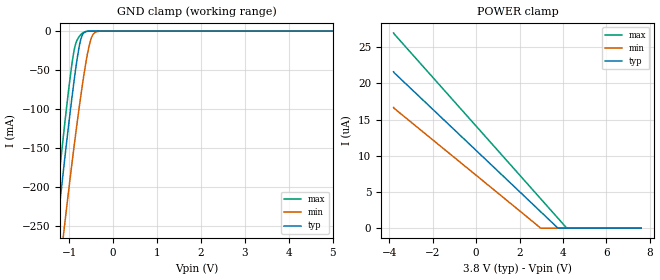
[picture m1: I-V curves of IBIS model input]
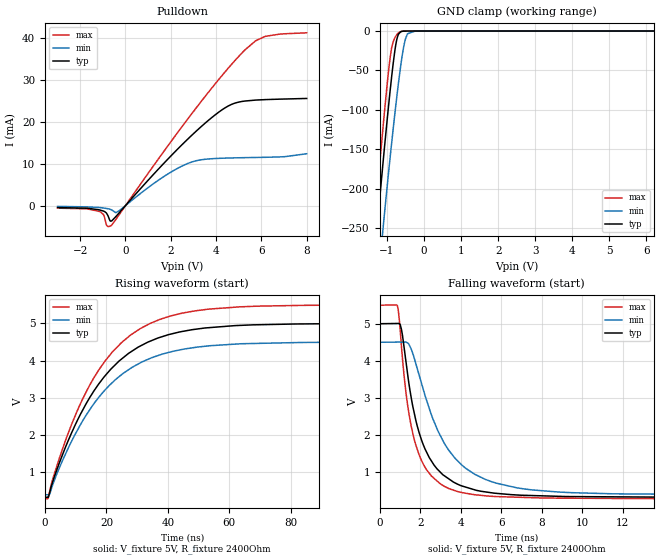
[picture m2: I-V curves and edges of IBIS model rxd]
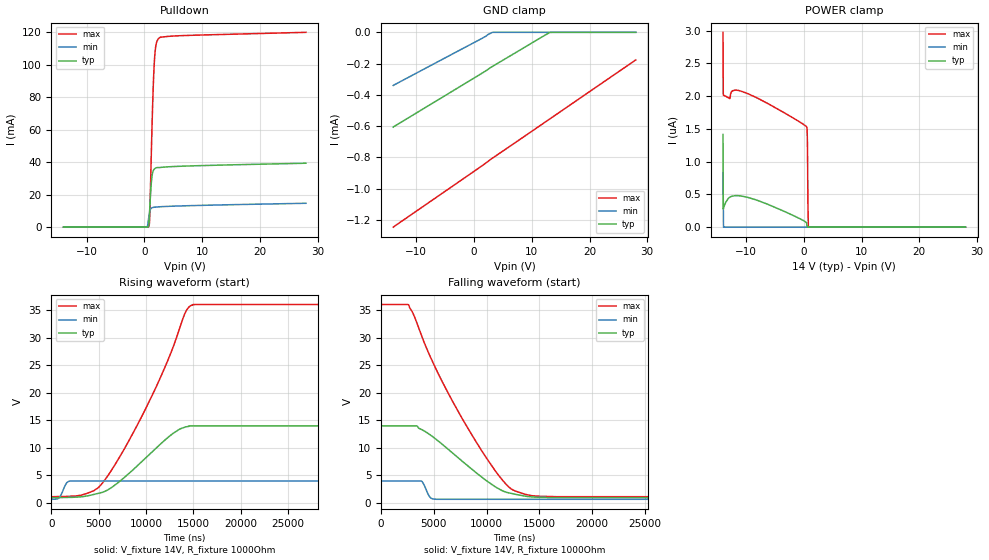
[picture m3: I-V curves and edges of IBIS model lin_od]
|Texas Instruments Incorporated
|TLIN1022-Q1 Dual Local Interconnect Network (LIN) Transceiver with Dominant
| State Timeout
[IBIS Ver]   4.1
[File name]   tlin1022-q1.ibs
[Date]   01/05/2018
[File Rev]   1.0
[Source]
| Texas Instruments Incorporated.
| Analog-eLab Design Center, HPA
| 12500 TI Blvd
| Dallas, TX -75243
[Notes]
| Rev 1.0: 01/05/2018
| - Initial version of the model
| - Model generated from simulations in SPECTRE
| - Model matched to SPICE simulation
| - C_comp although listed in numerical order of value are
|   obtained from varying PVT conditions. For PVT conditions for
|   each specific value refer the buffer description under
|   respective [Model]. IBIS model user is responsible for using
|   appropriate C_comp to simulate for Signal Integrity.
| - Warnings regarding combined Non-monotonicity of various models
|   have been reviewed and considered minor and can be ignored.
| - slow corner of lin_output model correlated for frequencies from 2KHz to 10KHz
[Disclaimer]
| This model is designed as an aid for customers of Texas Instruments.
| TI and its licensors and suppliers make no warranties, either expressed
| or implied, with respect to this  model, including the warranties of
| merchantability or fitness for a particular purpose. The model is
| provided solely on an "as is" basis. The entire risk as to its quality
| and performance is with the customer.
[Copyright]
(C) Copyright 2018 Texas Instruments Incorporated.All rights reserved.
|  Component TLIN1022DRQ1 14-pin SOIC - D package
|  Part # TLIN1022DRQ1
[Component]   TLIN1022DRQ1
[Manufacturer]  TI
[Package]   |14 SOIC - D package
|   typ   min   max
R_pkg   0.1   0.08   0.12
L_pkg   1.0nH   0.8nH   1.2nH
C_pkg   0.2pF   0.16pF   0.24pF
[Pin]  signal_name model_name   R_pin   L_pin   C_pin
1   RXD1   rxd   NA   NA   NA
2   EN1   input   NA   NA   NA
3   TXD1   input   NA   NA   NA
4   RXD2   rxd   NA   NA   NA
5   EN2   input   NA   NA   NA
6   NC   nc   NA   NA   NA
7   TXD2   input   NA   NA   NA
8   GND   gnd   NA   NA   NA
9   LIN2   lin   NA   NA   NA
10   VSUP   power   NA   NA   NA
11   NC   nc   NA   NA   NA
12   NC   nc   NA   NA   NA
13   LIN1   lin   NA   NA   NA
14   NC   nc   NA   NA   NA
|  Component TLIN1022DMTRQ1 14-pin VSON - DMT package
|  Part # TLIN1022DMTRQ1
[Component]   TLIN1022DMTRQ1
[Manufacturer]  TI
[Package]   |14 VSON - DMT package
|   typ   min   max
R_pkg   0   0   0
L_pkg   0   0   0
C_pkg   0   0   0
[Pin]  signal_name model_name   R_pin   L_pin   C_pin
1   RXD1   rxd   NA   NA   NA
2   EN1   input   NA   NA   NA
3   TXD1   input   NA   NA   NA
4   RXD2   rxd   NA   NA   NA
5   EN2   input   NA   NA   NA
6   NC   nc   NA   NA   NA
7   TXD2   input   NA   NA   NA
8   GND   gnd   NA   NA   NA
9   LIN2   lin   NA   NA   NA
10   VSUP   power   NA   NA   NA
11   NC   nc   NA   NA   NA
12   NC   nc   NA   NA   NA
13   LIN1   lin   NA   NA   NA
14   NC   nc   NA   NA   NA
|   Model Selectors
[Model Selector] lin
lin_od   14.0V   digital I/O_open_drain
lin_output   14.0V   digital Output
| Models and submodels in the file (4): input (Input), rxd (Open_sink), lin_od (I/O_open_drain), lin_output (Output)
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|   input Model
[Model]   input
Model_type   Input
Vinl = 0.8
Vinh = 2
|   typ   min   max
C_comp   3.46465E-12   3.07372E-12   4.01486E-12
| Where Nom  PVT is Nominal Process, 3.8V, 27C
|   Fast PVT is Strong Process,  4.2V, -55C
|   Slow PVT is Weak Process,   3V, 165C
[Voltage Range]   3.8   3   4.2
|Junction Temperature
[Temperature Range]   27   165   -55
[Power Clamp Reference]   3.8   3   4.2
[GND Clamp Reference]   0   0   0
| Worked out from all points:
|   GND clamp passes 1 mA (typ) near -0.63 V on its own axis
[GND Clamp]
|   Voltage   I(typ)   I(min)   I(max)
-3.8V     -1.716A    -1.741A    -1.714A
-1.417V   -329.7mA   -408.3mA   -288.7mA
-1.292V   -261.7mA   -342.8mA   -218.9mA
-1.269V   -249.6mA   -331mA     -206.5mA
-1.11V    -167.2mA   -250.8mA   -122.4mA
-904.4mV  -70.09mA   -154.5mA   -29.5mA
-847.4mV  -46.14mA   -129.4mA   -15.27mA
-767.6mV  -18.24mA   -95.69mA   -6.643mA
-665mV    -2.116mA   -55.77mA   -1.406mA
-494mV    -29.94uA   -8.423mA   -15.55uA
-300.2mV  -812.1nA   -88.71uA   -911.7nA
7.6V      0A         0A         0A
[POWER Clamp]
|   Voltage   I(typ)   I(min)   I(max)
-3.8V     21.6uA     16.67uA    26.97uA
2.96V     2.302uA    13.73nA    4.1uA
3.758V    23.08nA    0A         1.408uA
4.169V    0A         0A         15.11nA
7.6V      0A         0A         0A
|   rxd Model
[Model]   rxd
Model_type   Open_sink
Polarity   Non-Inverting
Vmeas = 2.5
Vref = 5
Cref = 2pF
Rref = 2400
|   typ   min   max
C_comp   3.72956E-12   3.27827E-12   4.2623E-12
| Where Nom  PVT is Nominal Process, 5V, 27C
|   Fast PVT is Strong Process,  5.5V, -55C
|   Slow PVT is Weak Process,   4.5V, 165C
[Voltage Range]   5   4.5   5.5
|Junction Temperature
[Temperature Range]   27   165   -55
[Pullup Reference]   5   4.5   5.5
[Pulldown Reference]   0   0   -0
[Power Clamp Reference]   5   4.5   5.5
[GND Clamp Reference]   0   0   0
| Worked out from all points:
|   slope of the pulldown table from 0 to 0.75 V, typ, clamps not added: 164 ohm
|   GND clamp passes 1 mA (typ) near -0.63 V on its own axis
|   falling waveform, V_fixture 5V, R_fixture 2400Ohm: 20-80 % time 1.33ns typ, 2.1ns min, 989ps max; typ from 5 V to 0.318 V
|   rising waveform, V_fixture 5V, R_fixture 2400Ohm: 20-80 % time 20.5ns typ, 20.7ns min, 20.1ns max; typ from 0.318 V to 5 V
[Pulldown]
|   Voltage   I(typ)   I(min)   I(max)
-3V       -478.7uA   -191.2uA   -603.9uA
-1.174V   -992.2uA   -450.9uA   -1.367mA
-965mV    -1.321mA   -581.3uA   -2.223mA
-844mV    -1.756mA   -677uA     -4.594mA
-646mV    -3.719mA   -938.5uA   -4.804mA
-426mV    -2.622mA   -1.694mA   -3.306mA
1.51V     9.031mA    6.263mA    11.55mA
2.841V    16.32mA    10.23mA    21.3mA
4.381V    23.25mA    11.31mA    31.77mA
5.283V    24.93mA    11.43mA    37.15mA
6.174V    25.26mA    11.51mA    40.34mA
8V        25.54mA    12.36mA    41.18mA
[GND Clamp]
|   Voltage   I(typ)   I(min)   I(max)
-3V       -1.245A    -1.286A    -1.23A
-1.559V   -408.7mA   -484.2mA   -369.9mA
-1.284V   -257.7mA   -339mA     -214.7mA
-1.086V   -155.7mA   -239.7mA   -110.7mA
-910mV    -72.76mA   -157.3mA   -31.65mA
-833mV    -40.68mA   -123.5mA   -13.39mA
-767mV    -18.25mA   -95.75mA   -6.8mA
-635mV    -1.061mA   -45.43mA   -766.8uA
-536mV    -90.64uA   -16.53mA   -55.21uA
-448mV    -8.124uA   -3.48mA    -2.688uA
-239mV    0A         -18.54uA   0A
8V        0A         0A         0A
[POWER Clamp]
|   Voltage   I(typ)   I(min)   I(max)
-3V       0A         0A         0A
0V        0A         0A         0A
8V        0A         0A         0A
[Ramp]
R_load = 2400
|   typ   min   max
dV/dt_r   2.80934/2.05464e-08   2.46843/2.06734e-08   3.13188/2.01086e-08
dV/dt_f   2.80935/1.32286e-09   2.46843/2.098e-09   3.13188/9.89047e-10
[Falling Waveform]
V_fixture = 5V
V_fixture_min = 4.5V
V_fixture_max = 5.5V
R_fixture = 2400Ohm
C_fixture = 0F
|   Time   V(typ)   V(min)   V(max)
0s        5V         4.5V       5.5V
877.3ps   5.007V     4.505V     5.486V
1.073ns   4.858V     4.506V     4.422V
1.389ns   3.611V     4.479V     2.779V
2.02ns    1.942V     3.48V      1.367V
2.871ns   1.064V     2.115V     740.3mV
4.079ns   620.7mV    1.177V     442.5mV
5.756ns   424.7mV    699.4mV    337.5mV
9.477ns   337.3mV    442.6mV    293.3mV
40ns      317.8mV    385.9mV    280.2mV
[Rising Waveform]
V_fixture = 5V
V_fixture_min = 4.5V
V_fixture_max = 5.5V
R_fixture = 2400Ohm
C_fixture = 0F
|   Time   V(typ)   V(min)   V(max)
0s        317.8mV    385.9mV    280.2mV
943.3ps   319.6mV    384.8mV    279.9mV
1.502ns   449.3mV    398.4mV    480.9mV
6.576ns   1.653V     1.468V     1.83V
11.47ns   2.545V     2.266V     2.829V
15.68ns   3.152V     2.812V     3.505V
21.94ns   3.811V     3.409V     4.233V
34.19ns   4.521V     4.058V     5V
53.07ns   4.885V     4.395V     5.385V
600ns     5V         4.5V       5.5V
|   lin_od Model
[Model]   lin_od
Model_type   I/O_open_drain
Polarity   Non-Inverting
Enable   Active-High
Vinl = 5.6
Vinh = 8.4
Vmeas = 7
Vref = 14
Cref = 2pF
Rref = 1000
|   typ   min   max
C_comp   3.52891E-11   3.03138E-11   3.67824E-11
[Model spec]
|subparameter
Vinl   5.6   1.6   14.4
Vinh   8.4   2.4   21.6
| Where Nom  PVT is Nominal Process, 14V, 27C
|   Fast PVT is Strong Process,  36V, -55C
|   Slow PVT is Weak Process,   4V, 165C
[Voltage Range]   14   4   36
|Junction Temperature
[Temperature Range]   27   165   -55
[Pullup Reference]   14   4   36
[Pulldown Reference]   -0   0   0
[Power Clamp Reference]   14   4   36
[GND Clamp Reference]   0   0   0
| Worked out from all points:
|   slope of the pulldown table from 0 to 2.1 V, typ, clamps not added: 57.4 ohm
|   falling waveform, V_fixture 14V, R_fixture 1000Ohm: 20-80 % time 5.03us typ, 474ns min, 5.9us max; typ from 14 V to 0.965 V
|   rising waveform, V_fixture 14V, R_fixture 1000Ohm: 20-80 % time 5.02us typ, 519ns min, 5.89us max; typ from 0.965 V to 14 V
[Pulldown]
|   Voltage   I(typ)   I(min)   I(max)
-14V      1.08pA     612pA      13.5pA
364mV     441nA      18.12uA    299.7nA
574mV     11.79uA    1.259mA    3.225uA
784mV     1.915mA    6.519mA    677.8uA
868mV     6.608mA    8.41mA     2.059mA
952mV     12.48mA    9.825mA    8.527mA
1.204V    27.17mA    11.68mA    44.78mA
1.414V    33.19mA    12.07mA    72.61mA
1.708V    35.71mA    12.27mA    100.2mA
2.002V    36.45mA    12.38mA    111.9mA
2.59V     36.72mA    12.53mA    116.6mA
28V       39.38mA    14.71mA    120mA
[GND Clamp]
|   Voltage   I(typ)   I(min)   I(max)
-14V      -606uA     -340uA     -1.246mA
3.178V    -218.1uA   -283.1nA   -804.7uA
13.17V    -69.03nA   0A         -552.4uA
28V       0A         0A         -176.6uA
[POWER Clamp]
|   Voltage   I(typ)   I(min)   I(max)
-14V      1.413uA    828.1nA    2.973uA
-13.96V   279.3nA    414nA      2.015uA
-13.92V   292.2nA    0A         2.013uA
-12.7V    463.9nA    0A         2.032uA
-10.14V   463.5nA    0A         2.052uA
490mV     55.92nA    0A         1.53uA
574mV     13.16nA    0A         1.463uA
616mV     0A         0A         1.301uA
658mV     0A         0A         940.7nA
700mV     0A         0A         391.4nA
784mV     0A         0A         0A
28V       0A         0A         0A
[Ramp]
R_load = 1000
|   typ   min   max
dV/dt_r   7.82063/5.02021e-06   2/5.13924e-07   20.9135/5.88986e-06
dV/dt_f   7.82062/5.01724e-06   2.00001/4.72315e-07   20.9135/5.90389e-06
[Falling Waveform]
V_fixture = 14V
V_fixture_min = 4V
V_fixture_max = 36V
R_fixture = 1000Ohm
C_fixture = 0F
|   Time   V(typ)   V(min)   V(max)
0s        14V        4V         36V
2.61us    14V        4V         35.94V
3.836us   13.32V     3.955V     30.35V
4.506us   12.55V     1.395V     27.18V
4.872us   12.05V     748.7mV    25.65V
7.553us   7.803V     675mV      15.77V
10.82us   2.949V     674.3mV    5.849V
12.65us   1.615V     673.9mV    2.231V
16.23us   998.6mV    673.2mV    1.162V
50us      964.9mV    666.4mV    1.142V
[Rising Waveform]
V_fixture = 14V
V_fixture_min = 4V
V_fixture_max = 36V
R_fixture = 1000Ohm
C_fixture = 0F
|   Time   V(typ)   V(min)   V(max)
0s        964.9mV    666.4mV    1.142V
858.5ns   990mV      1.033V     1.167V
1.893us   1.02V      3.966V     1.214V
4.463us   1.547V     3.992V     2.21V
5.836us   2.276V     3.992V     4.639V
9.963us   8.187V     3.993V     17.14V
12.3us    11.88V     3.993V     25.9V
14.14us   13.78V     3.994V     34.55V
14.95us   13.99V     3.994V     35.98V
50us      14V        4V         36V
